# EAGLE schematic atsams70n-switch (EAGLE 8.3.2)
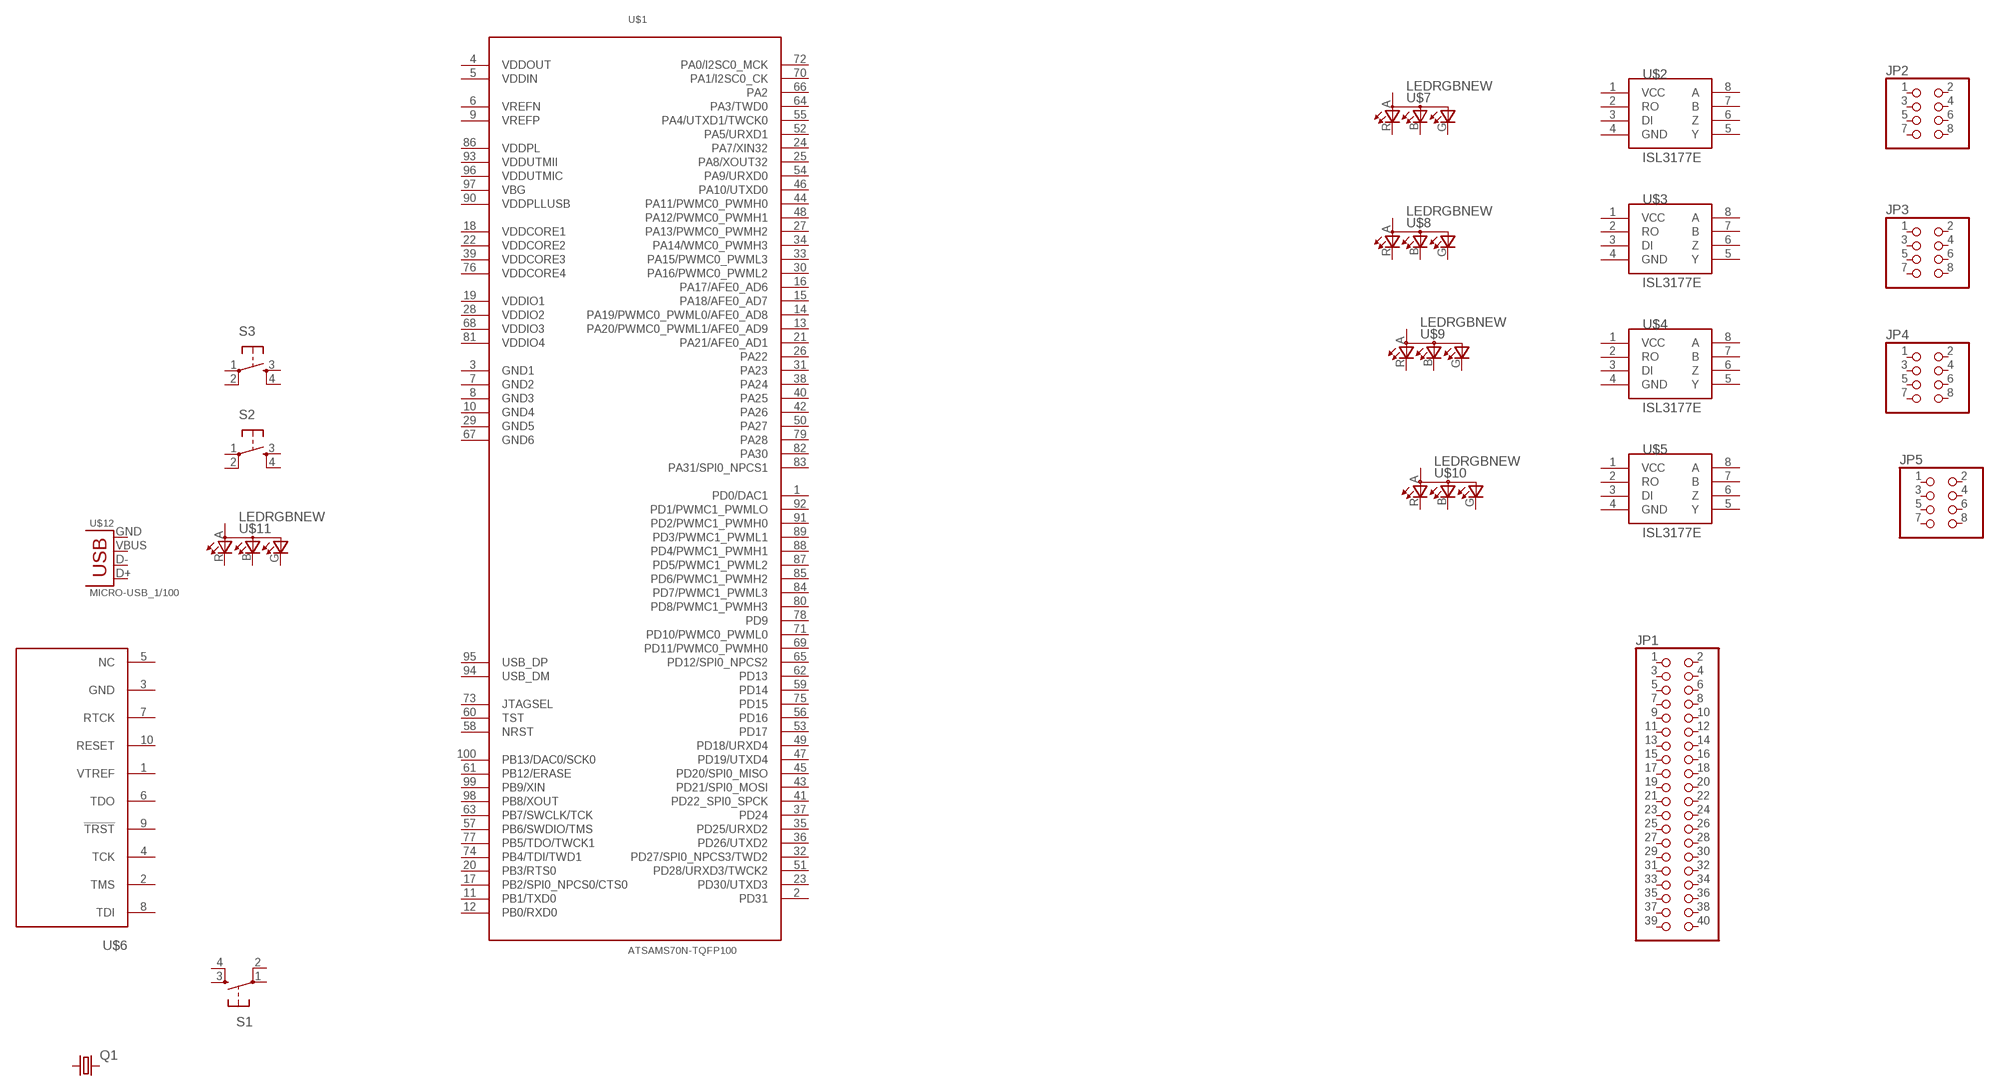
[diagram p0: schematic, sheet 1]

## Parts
JP1  PINHD-2X20  [2X20]
JP2  PINHD-2X4  [2X04]
JP3  PINHD-2X4  [2X04]
JP4  PINHD-2X4  [2X04]
JP5  PINHD-2X4  [2X04]
Q1  CRYSTALCTS406  [CTS406]
S1  6MM_SWITCH6MM_SWITCH  [6MM_SWITCH]
S2  6MM_SWITCH6MM_SWITCH  [6MM_SWITCH]
S3  6MM_SWITCH6MM_SWITCH  [6MM_SWITCH]
U$1  ATSAMS70N-TQFP100  [TQFP100-14X14]
U$2  ISL3177E  [MSOP8]
U$3  ISL3177E  [MSOP8]
U$4  ISL3177E  [MSOP8]
U$5  ISL3177E  [MSOP8]
U$6  TC2050-MCP-NL  [TC2030-MCP-NL]
U$7  LEDRGBNEW  [P-LCC-4]
U$8  LEDRGBNEW  [P-LCC-4]
U$9  LEDRGBNEW  [P-LCC-4]
U$10  LEDRGBNEW  [P-LCC-4]
U$11  LEDRGBNEW  [P-LCC-4]
U$12  MICRO-USB_1/100  [DX4R005HJ5_100]
Unconnected: JP1.1 JP1.2 JP1.3 JP1.4 JP1.5 JP1.6 JP1.7 JP1.8 JP1.9 JP1.10 JP1.11 JP1.12 JP1.13 JP1.14 JP1.15 JP1.16 JP1.17 JP1.18 JP1.19 JP1.20 JP1.21 JP1.22 JP1.23 JP1.24 JP1.25 JP1.26 JP1.27 JP1.28 JP1.29 JP1.30 JP1.31 JP1.32 JP1.33 JP1.34 JP1.35 JP1.36 JP1.37 JP1.38 JP1.39 JP1.40 JP2.1 JP2.2 JP2.3 JP2.4 JP2.5 JP2.6 JP2.7 JP2.8 JP3.1 JP3.2 JP3.3 JP3.4 JP3.5 JP3.6 JP3.7 JP3.8 JP4.1 JP4.2 JP4.3 JP4.4 JP4.5 JP4.6 JP4.7 JP4.8 JP5.1 JP5.2 JP5.3 JP5.4 JP5.5 JP5.6 JP5.7 JP5.8 Q1.1 Q1.3 S1.1(P) S1.2(P1) S1.3(S) S1.4(S1) S2.1(P) S2.2(P1) S2.3(S) S2.4(S1) S3.1(P) S3.2(P1) S3.3(S) S3.4(S1) U$1.1(PD0/DAC1) U$1.2(PD31) U$1.3(GND1) U$1.4(VDDOUT) U$1.5(VDDIN) U$1.6(VREFN) U$1.7(GND2) U$1.8(GND3) U$1.9(VREFP) U$1.10(GND4) U$1.11(PB1/TXD0) U$1.12(PB0/RXD0) U$1.13(PA20/PWMC0_PWML1/AFE0_AD9) U$1.14(PA19/PWMC0_PWML0/AFE0_AD8) U$1.15(PA18/AFE0_AD7) U$1.16(PA17/AFE0_AD6) U$1.17(PB2/SPI0_NPCS0/CTS0) U$1.18(VDDCORE1) U$1.19(VDDIO1) U$1.20(PB3/RTS0) U$1.21(PA21/AFE0_AD1) U$1.22(VDDCORE2) U$1.23(PD30/UTXD3) U$1.24(PA7/XIN32) U$1.25(PA8/XOUT32) U$1.26(PA22) U$1.27(PA13/PWMC0_PWMH2) U$1.28(VDDIO2) U$1.29(GND5) U$1.30(PA16/PWMC0_PWML2) U$1.31(PA23) U$1.32(PD27/SPI0_NPCS3/TWD2) U$1.33(PA15/PWMC0_PWML3) U$1.34(PA14/WMC0_PWMH3) U$1.35(PD25/URXD2) U$1.36(PD26/UTXD2) U$1.37(PD24) U$1.38(PA24) U$1.39(VDDCORE3) U$1.40(PA25) U$1.41(PD22_SPI0_SPCK) U$1.42(PA26) U$1.43(PD21/SPI0_MOSI) U$1.44(PA11/PWMC0_PWMH0) U$1.45(PD20/SPI0_MISO) U$1.46(PA10/UTXD0) U$1.47(PD19/UTXD4) U$1.48(PA12/PWMC0_PWMH1) U$1.49(PD18/URXD4) U$1.50(PA27) U$1.51(PD28/URXD3/TWCK2) U$1.52(PA5/URXD1) U$1.53(PD17) U$1.54(PA9/URXD0) U$1.55(PA4/UTXD1/TWCK0) U$1.56(PD16) U$1.57(PB6/SWDIO/TMS) U$1.58(NRST) U$1.59(PD14) U$1.60(TST) U$1.61(PB12/ERASE) U$1.62(PD13) U$1.63(PB7/SWCLK/TCK) U$1.64(PA3/TWD0) U$1.65(PD12/SPI0_NPCS2) U$1.66(PA2) U$1.67(GND6) U$1.68(VDDIO3) U$1.69(PD11/PWMC0_PWMH0) U$1.70(PA1/I2SC0_CK) U$1.71(PD10/PWMC0_PWML0) U$1.72(PA0/I2SC0_MCK) U$1.73(JTAGSEL) U$1.74(PB4/TDI/TWD1) U$1.75(PD15) U$1.76(VDDCORE4) U$1.77(PB5/TDO/TWCK1) U$1.78(PD9) U$1.79(PA28) U$1.80(PD8/PWMC1_PWMH3) U$1.81(VDDIO4) U$1.82(PA30) U$1.83(PA31/SPI0_NPCS1) U$1.84(PD7/PWMC1_PWML3) U$1.85(PD6/PWMC1_PWMH2) U$1.86(VDDPL) U$1.87(PD5/PWMC1_PWML2) U$1.88(PD4/PWMC1_PWMH1) U$1.89(PD3/PWMC1_PWML1) U$1.90(VDDPLLUSB) U$1.91(PD2/PWMC1_PWMH0) U$1.92(PD1/PWMC1_PWMLO) U$1.93(VDDUTMII) U$1.94(USB_DM) U$1.95(USB_DP) U$1.96(VDDUTMIC) U$1.97(VBG) U$1.98(PB8/XOUT) U$1.99(PB9/XIN) U$1.100(PB13/DAC0/SCK0) U$2.1(VCC) U$2.2(RO) U$2.3(DI) U$2.4(GND) U$2.5(Y) U$2.6(Z) U$2.7(B) U$2.8(A) U$3.1(VCC) U$3.2(RO) U$3.3(DI) U$3.4(GND) U$3.5(Y) U$3.6(Z) U$3.7(B) U$3.8(A) U$4.1(VCC) U$4.2(RO) U$4.3(DI) U$4.4(GND) U$4.5(Y) U$4.6(Z) U$4.7(B) U$4.8(A) U$5.1(VCC) U$5.2(RO) U$5.3(DI) U$5.4(GND) U$5.5(Y) U$5.6(Z) U$5.7(B) U$5.8(A) U$6.1(VTREF) U$6.2(TMS) U$6.3(GND) U$6.4(TCK) U$6.5(NC) U$6.6(TDO) U$6.7(RTCK) U$6.8(TDI) U$6.9(!TRST) U$6.10(RESET) U$7.A(A2) U$7.B(CBLUE) U$7.G(CGREEN) U$7.R(CRED) U$8.A(A2) U$8.B(CBLUE) U$8.G(CGREEN) U$8.R(CRED) U$9.A(A2) U$9.B(CBLUE) U$9.G(CGREEN) U$9.R(CRED) U$10.A(A2) U$10.B(CBLUE) U$10.G(CGREEN) U$10.R(CRED) U$11.A(A2) U$11.B(CBLUE) U$11.G(CGREEN) U$11.R(CRED) U$12.D+ U$12.D- U$12.GND U$12.VBUS

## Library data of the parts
JP1 = pinhead:PINHD-2X20: PIN HEADER
JP2-JP5 = pinhead:PINHD-2X4: PIN HEADER
Q1 = crystal:CRYSTAL: CRYSTAL; OC_FARNELL: unknown; OC_NEWARK: unknown
S1-S3 = fab:6MM_SWITCH: OMRON SWITCH
U$1 = fab:ATSAMS70N-TQFP100
U$2-U$5 = fab:ISL3177E
U$6 = tag-connect-2050:TC2050: TAG-CONNECT ISP Connector Manufacturer: Tag-Connect Cable for easy In-Circuit PCB Programming. Designed for JTAG 10 pin, suitable for many others. Pin Connection for TC2050 NL. PADDescription 1VTREF 2TMS 3GND 4TCK 5NC 6TDO 7RTCK 8TDI 9!TRST 10RESET ©2009 ROFA.cz Modified 7/2011 by Tim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
U$7-U$11 = fab:LEDRGBNEW
U$12 = fab:MICRO-USB: SMD micro USB connector as found in the fablab inventory. Three footprint variants included: original, as described by manufacturer's datasheet for milling with the 1/100" bit for milling with the 1/64" bit Made by Zaerc.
